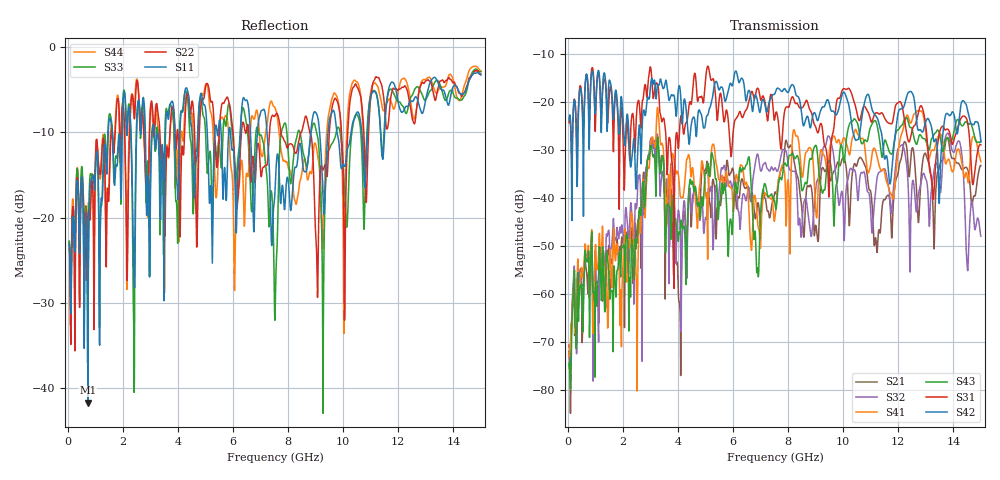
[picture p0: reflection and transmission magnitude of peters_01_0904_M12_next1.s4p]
# MHZ S RI R 50.00
! FREQ  S11  S12  S13  S14
!  S21  S22  S23  S24
!  S31  S32  S33  S34
!  S41  S42  S43  S44
!  REAL  IMAG  REAL  IMAG  REAL  IMAG  REAL  IMAG
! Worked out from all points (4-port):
!   1496 points, 50 MHz to 15 GHz, reference 50 ohm
!   strongest paths, dB at 50 MHz, 3.79 GHz, 7.53 GHz, 11.27 GHz, 15 GHz:
!     S42: -23.8, -18.6, -18.1, -23.8, -28.4
!     S31: -24.3, -32.6, -23.1, -22.4, -28.9
!     S43: -74.4, -40.3, -41.4, -26.0, -28.1
!     S41: -73.0, -30.9, -43.5, -32.4, -32.5
!     S32: -71.1, -33.4, -33.7, -35.0, -48.0
!     S21: -72.0, -42.1, -38.8, -47.9, -33.3
!   lowest |S11| = -41.7 dB at 730 MHz (marker M1), VSWR 1.02, Z = 49.5 + j0.676 ohm
!   |S11| at or under -10 dB: start of sweep to 1.47 GHz; 7.235 GHz to 8.824 GHz (1.589 GHz wide, 19.8 % of centre); 9.773 GHz to 10.29 GHz (514.8 MHz wide, 5.13 % of centre)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
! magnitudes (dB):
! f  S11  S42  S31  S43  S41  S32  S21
! 50 MHz  -23.1  -23.8  -24.3  -74.4  -73.0  -71.1  -72.0
! 730 MHz  -41.7  -16.9  -16.1  -53.1  -51.5  -52.2  -59.9
! 2.49 GHz  -11.6  -37.3  -23.3  -49.5  -57.6  -42.2  -48.8
! 3.27 GHz  -10.1  -16.4  -16.5  -27.3  -21.5  -27.2  -28.1
! 4.06 GHz  -11.3  -16.7  -25.8  -47.3  -38.0  -44.2  -62.1
! 5.02 GHz  -7.8  -23.7  -14.3  -34.8  -39.5  -44.4  -33.8
! 15 GHz  -3.3  -28.4  -28.9  -28.1  -32.5  -48.0  -33.3
